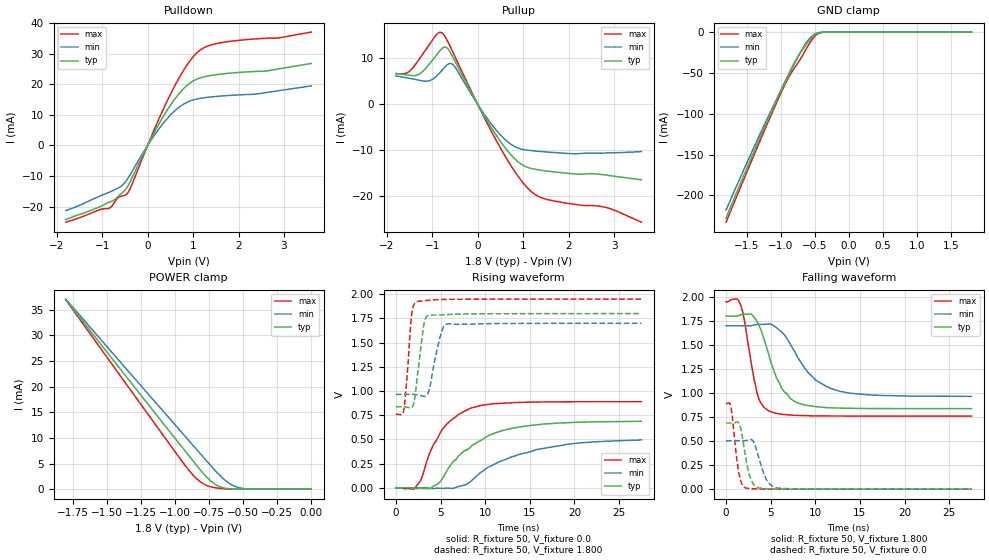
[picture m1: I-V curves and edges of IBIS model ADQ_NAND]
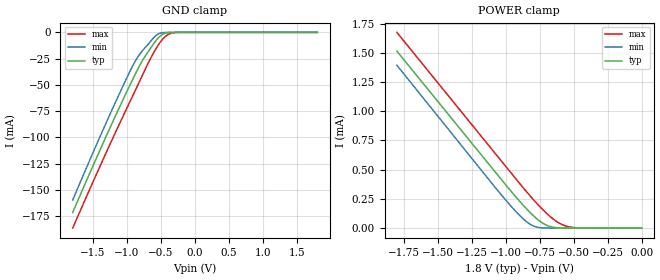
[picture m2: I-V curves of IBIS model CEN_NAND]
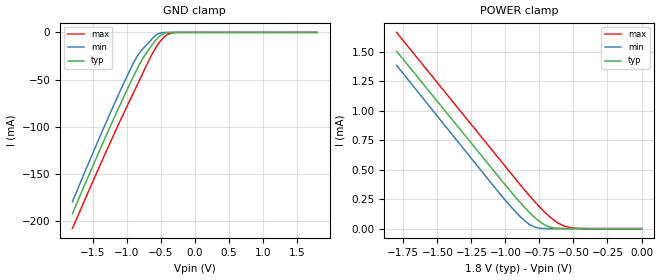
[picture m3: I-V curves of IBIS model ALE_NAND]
| This IBIS file was created by s2ibis3 version 1.1
| North Carolina State University, ERL, 2006
[IBIS ver] 3.2
[File name] s34ms04g1_t_i_18_r2.ibs
[File Rev] 2.0
|   Rev1.0 Initial release with updated measurement
|   (X8 LEGACY/ONFI F41 98462AD 41061)
|   Rev2.0 Update 0A for 0V
[Date] 7/23/2014
[Source] Spansion IBIS team
|   Email: dl.ibisteam@spansion.com
[Notes]  Generated IBIS models from SPICE simulations.
|   VIO=1.65V - 1.95V, Temperature Range: Industrial (-40oC to +90oC).
[Disclaimer] THE MODEL LIBRARIES ARE PROVIDED AS IS.
[Copyright] (C) COPYRIGHT 2014
| SPANSION LLC
| ALL RIGHTS RESERVED.
|   Component S34MS04G1 X8 LEGACY/ONFI F41 in TSOP48 package
[Component]   S34MS04G1
[Manufacturer]   Spansion
[Package]
| variable   typ   min   max
R_pkg   146.31mOhm   135.08mOhm   174.84mOhm
L_pkg   9.54nH   5.88nH   15.8nH
C_pkg   0.80pF   0.42pF   2.25pF
[Pin]   signal_name   model_name   R_pin   L_pin   C_pin
1   NC   NC
2   NC   NC
3   NC   NC
4   NC   NC
5   NC   NC
6   NC   NC
7   R/B#   RB_NAND   135.60m   7.62n   2.25p
8   RE   REN_NAND   135.66m   15.5n   0.81p
9   CE   CEN_NAND   135.08m   15.8n   0.80p
10   NC   NC
11   NC   NC
12   VCC   POWER
13   VSS   GND
14   NC   NC
15   NC   NC
16   CLE   CLE_NAND   138.23m   15.8n   0.81p
17   ALE   ALE_NAND   142.47m   15.6n   0.82p
18   WE   WEN_NAND   146.37m   12.0n   0.91p
19   WP   WP_NAND   149.93m   9.29n   1.93p
20   NC   NC
21   NC   NC
22   NC   NC
23   NC   NC
24   NC   NC
25   NC   NC
26   NC   NC
27   NC   NC
28   NC   NC
29   IO0   ADQ_NAND   174.84m   6.38n   0.46p
30   IO1   ADQ_NAND   167.68m   6.29n   0.46p
31   IO2   ADQ_NAND   161.34m   6.93n   0.45p
32   IO3   ADQ_NAND   155.11m   6.74n   0.44p
33   NC   NC
34   NC   NC
35   NC   NC
36   VSS   GND
37   VCC   POWER
38   NC   NC
39   NC   NC
40   NC   NC
41   IO4   ADQ_NAND   136.94m   6.48n   0.42p
42   IO5   ADQ_NAND   136.82m   6.60n   0.42p
43   IO6   ADQ_NAND   139.20m   5.88n   0.43p
44   IO7   ADQ_NAND   139.40m   5.92n   0.43p
45   NC   NC
46   NC   NC
47   NC   NC
48   NC   NC
| Models and submodels in the file (8): ADQ_NAND (I/O), CEN_NAND (Input), ALE_NAND (Input), CLE_NAND (Input), WEN_NAND (Input), REN_NAND (Input), WP_NAND (Input), RB_NAND (Open_drain)
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|   Model ADQ_NAND
[Model]   ADQ_NAND
Model_type   I/O
Polarity   Non-Inverting
Enable   Active-High
Vinl   = 0.360V
Vinh   = 1.440V
Vmeas  = 0.900V
Vref   = 0.900V
Rref   = 8350ohm
Cref   = 30pF
| variable   typ   min   max
C_comp   3.72pF   3.35pF   4.46pF
| variable   typ   min   max
[Temperature Range]  25.00   85.00   -30.00
[Voltage Range]   1.800   1.700   1.950
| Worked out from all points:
|   slope of the pulldown table from 0 to 0.27 V, typ, clamps not added: 35.8 ohm
|   slope of the pullup table from 0 to 0.27 V, typ, clamps not added: 58.9 ohm
|   GND clamp passes 1 mA (typ) near -0.44 V on its own axis
|   POWER clamp passes 1 mA (typ) near -0.71 V on its own axis
|   rising waveform, R_fixture 50, V_fixture 0.0: 20-80 % time 5.18ns typ, 7.01ns min, 3.23ns max; typ from 0 V to 0.687 V
|   falling waveform, R_fixture 50, V_fixture 1.800: 20-80 % time 2.28ns typ, 3.54ns min, 1.35ns max; typ from 1.8 V to 0.838 V
|   rising waveform, R_fixture 50, V_fixture 1.800: 20-80 % time 754ps typ, 979ps min, 578ps max; typ from 0.838 V to 1.8 V
|   falling waveform, R_fixture 50, V_fixture 0.0: 20-80 % time 849ps typ, 1.08ns min, 665ps max; typ from 0.688 V to 0 V
[Pulldown]
| voltage   I(typ)   I(min)   I(max)
-1.8V     -24.24mA   -21.3mA    -25.1mA
-828mV    -18.44mA   -15.22mA   -20.42mA
-666mV    -16.9mA    -14.08mA   -17.25mA
-450mV    -13.69mA   -11.16mA   -15.84mA
-342mV    -10.59mA   -8.492mA   -12.67mA
90mV      2.627mA    2.052mA    3.223mA
468mV     12.38mA    9.368mA    15.7mA
792mV     18.59mA    13.51mA    24.57mA
1.116V    21.88mA    15.27mA    30.73mA
1.602V    23.31mA    16.14mA    33.56mA
2.628V    24.38mA    17.33mA    35.06mA
3.6V      26.82mA    19.46mA    37.06mA
[Pullup]
| voltage   I(typ)   I(min)   I(max)
-1.8V     6.711mA    6.204mA    6.703mA
-1.53V    6.378mA    5.733mA    7.009mA
-1.314V   6.462mA    5.32mA     9.487mA
-1.044V   9.028mA    5.211mA    13.32mA
-774mV    12.29mA    7.564mA    15.5mA
-558mV    10.5mA     8.79mA     11.62mA
468mV     -7.609mA   -6.274mA   -8.926mA
792mV     -11.62mA   -9.059mA   -14.28mA
1.116V    -13.78mA   -9.986mA   -18.39mA
1.494V    -14.47mA   -10.34mA   -20.6mA
2.844V    -15.42mA   -10.57mA   -22.48mA
3.6V      -16.4mA    -10.26mA   -25.64mA
[GND_clamp]
| voltage   I(typ)   I(min)   I(max)
-1.8V     -227.8mA   -218mA     -232.8mA
-1.44V    -155.9mA   -150mA     -160.5mA
-1.152V   -100.6mA   -98.3mA    -104.1mA
-972mV    -67.31mA   -67.55mA   -70.33mA
-864mV    -48.19mA   -49.77mA   -52.81mA
-756mV    -31.2mA    -32.3mA    -39.05mA
-612mV    -13.69mA   -11.59mA   -18.85mA
-540mV    -6.376mA   -4.919mA   -9.319mA
-468mV    -1.892mA   -1.445mA   -2.895mA
-396mV    -317.5uA   -280.6uA   -453uA
-324mV    -33.8uA    -40.79uA   -36.53uA
1.8V      190.5pA    3.644nA    114.8pA
[POWER_clamp]
| voltage   I(typ)   I(min)   I(max)
-1.8V     36.95mA    37.04mA    36.91mA
-936mV    7.811mA    10.64mA    5.005mA
-864mV    5.405mA    8.449mA    2.668mA
-810mV    3.633mA    6.808mA    1.367mA
-738mV    1.629mA    4.621mA    470.5uA
-684mV    632.8uA    3.05mA     201.6uA
-612mV    108.6uA    1.346mA    45.35uA
-540mV    13.14uA    364uA      4.716uA
-432mV    393.1nA    23.68uA    63.01nA
0V        0A         0A         0A
[Ramp]
| variable   typ   min   max
dV/dt_r   412.33m/5.13n   297.56m/6.78n   534.08m/3.12n
dV/dt_f   577.47m/2.21n   440.84m/3.34n   713.83m/1.33n
R_load = 50
[Rising Waveform]
R_fixture = 50
V_fixture = 0.0
| time   V(typ)   V(min)   V(max)
0s        35.16uV    -178.1nV   566.9uV
2.14ns    -6.557mV   130.9uV    -3.442mV
2.788ns   -6.033mV   243.2uV    79.41mV
3.724ns   -9.674mV   -3.583mV   345.6mV
5.02ns    69.11mV    -5.603mV   578.2mV
6.388ns   268.6mV    -6.468mV   712.1mV
8.224ns   410.3mV    54.63mV    818.5mV
11.14ns   567mV      250.5mV    869.2mV
15.57ns   649.1mV    391.9mV    885.1mV
27.5ns    686.7mV    494.2mV    890.1mV
[Falling Waveform]
R_fixture   = 50
V_fixture   = 1.800
V_fixture_min = 1.700
V_fixture_max = 1.950
| time   V(typ)   V(min)   V(max)
0s        1.8V       1.7V       1.949V
1.636ns   1.814V     1.7V       1.915V
2.788ns   1.823V     1.701V     1.33V
3.508ns   1.738V     1.713V     991.1mV
4.804ns   1.395V     1.718V     813.9mV
6.136ns   1.063V     1.643V     780.5mV
7.108ns   950.1mV    1.523V     772mV
9.124ns   870.7mV    1.22V      764mV
11.61ns   846.8mV    1.052V     761.3mV
27.5ns    837.6mV    965.4mV    760.3mV
[Rising Waveform]
R_fixture   = 50
V_fixture   = 1.800
V_fixture_min = 1.700
V_fixture_max = 1.950
| time   V(typ)   V(min)   V(max)
0s        837.5mV    965.1mV    760.9mV
880ps     837.4mV    965.1mV    802.3mV
1.744ns   827.2mV    966mV      1.774V
2.068ns   900.2mV    964.8mV    1.901V
2.356ns   1.119V     961.3mV    1.923V
3.328ns   1.752V     947.4mV    1.934V
3.76ns    1.784V     1.024V     1.939V
5.02ns    1.785V     1.582V     1.945V
5.632ns   1.789V     1.689V     1.946V
27.5ns    1.8V       1.7V       1.95V
[Falling Waveform]
R_fixture = 50
V_fixture = 0.0
| time   V(typ)   V(min)   V(max)
0s        688.2mV    503.8mV    890.1mV
556ps     688mV      503.8mV    846.1mV
1.42ns    690.5mV    503.7mV    174.4mV
1.744ns   583.4mV    503.6mV    58.33mV
2.176ns   344.4mV    505.6mV    13.62mV
2.572ns   163.6mV    514.1mV    7.024mV
3.112ns   45.85mV    484.8mV    3.77mV
4.48ns    5.218mV    106.9mV    1.058mV
5.56ns    2.061mV    15.63mV    502.1uV
27.5ns    -1.069uV   450.8nV    -607.7nV
|   Model CEN_NAND
[Model]   CEN_NAND
Model_type   Input
Vinl = 0.360V
Vinh = 1.440V
| variable   typ   min   max
C_comp   2.20pF   1.98pF   2.64pF
| variable   typ   min   max
[Temperature Range]  25.00   -30.00   85.00
[Voltage Range]   1.800   1.700   1.950
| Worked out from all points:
|   GND clamp passes 1 mA (typ) near -0.44 V on its own axis
|   POWER clamp passes 1 mA (typ) near -1.44 V on its own axis
[GND_clamp]
| voltage   I(typ)   I(min)   I(max)
-1.8V     -171.6mA   -159.8mA   -186.5mA
-1.296V   -97.42mA   -84.54mA   -113mA
-1.044V   -62mA      -48.92mA   -77.85mA
-900mV    -42.52mA   -29.89mA   -58.24mA
-828mV    -33.22mA   -22.07mA   -48.35mA
-756mV    -24.99mA   -16.18mA   -38.4mA
-612mV    -11.15mA   -5.36mA    -19.76mA
-504mV    -3.085mA   -583.3uA   -8.654mA
-432mV    -700.3uA   -55.3uA    -3.629mA
-360mV    -93.93uA   -2.943uA   -1.015mA
-252mV    -2.155uA   -17.44nA   -71.47uA
1.8V      140.8pA    79.49pA    15.92nA
[POWER_clamp]
| voltage   I(typ)   I(min)   I(max)
-1.8V     1.514mA    1.393mA    1.674mA
-1.026V   408.5uA    277uA      566.8uA
-900mV    234.3uA    112.6uA    386.8uA
-828mV    143.4uA    39.7uA     287.2uA
-774mV    83.73uA    9.844uA    216.3uA
-702mV    26.55uA    788.6nA    130.1uA
-630mV    4.495uA    62.15nA    60.75uA
-558mV    538.1nA    3.703nA    18.71uA
-450mV    16.7nA     132.3pA    1.525uA
0V        0A         0A         0A
|   Model ALE_NAND
[Model]   ALE_NAND
Model_type   Input
Vinl = 0.360V
Vinh = 1.440V
| variable   typ   min   max
C_comp   2.20pF   1.98pF   2.64pF
| variable   typ   min   max
[Temperature Range]  25.00   -30.00   85.00
[Voltage Range]   1.800   1.700   1.950
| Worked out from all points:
|   GND clamp passes 1 mA (typ) near -0.44 V on its own axis
|   POWER clamp passes 1 mA (typ) near -1.44 V on its own axis
[GND_clamp]
| voltage   I(typ)   I(min)   I(max)
-1.8V     -192.3mA   -179.6mA   -208.1mA
-1.26V    -102.4mA   -88.17mA   -119.4mA
-1.008V   -62.69mA   -48.22mA   -80.06mA
-864mV    -41.05mA   -27.42mA   -58.29mA
-756mV    -26.47mA   -16.77mA   -41.79mA
-648mV    -15.24mA   -8.416mA   -25.81mA
-576mV    -8.287mA   -3.156mA   -16.52mA
-504mV    -3.152mA   -587.1uA   -8.981mA
-432mV    -704.7uA   -55.34uA   -3.704mA
-360mV    -94.01uA   -2.944uA   -1.022mA
-252mV    -2.155uA   -17.44nA   -71.51uA
1.8V      140.8pA    79.49pA    15.92nA
[POWER_clamp]
| voltage   I(typ)   I(min)   I(max)
-1.8V     1.507mA    1.387mA    1.667mA
-1.026V   406.6uA    275.7uA    564.2uA
-900mV    233.3uA    112.2uA    385.1uA
-828mV    142.8uA    39.6uA     285.9uA
-774mV    83.46uA    9.834uA    215.4uA
-702mV    26.5uA     788.5nA    129.7uA
-630mV    4.493uA    62.15nA    60.59uA
-558mV    538.1nA    3.703nA    18.69uA
-450mV    16.7nA     132.3pA    1.525uA
0V        0A         0A         0A
